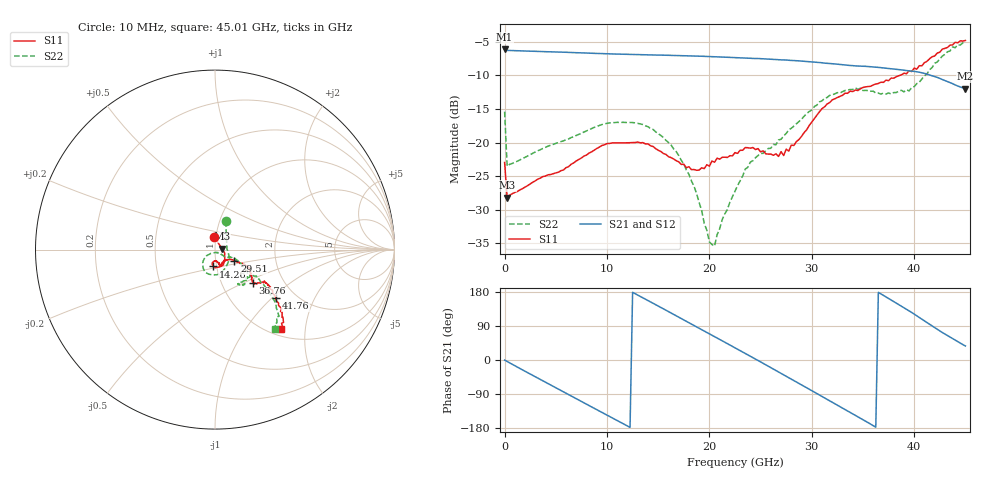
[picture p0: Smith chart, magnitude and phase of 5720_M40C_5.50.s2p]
! Device:  ADRF5720
! Description: 0.5dB LSB GaAs MMIC 6-bit Digital Attenuator
! Frequency:  0.000009 -  40 GHz
! Ports:
!	RF1	= Port 1
!	RF2	= Port 2
! Vdd:  3.3 Volt
! Vss:  -3.3 Volt
! Control:  0/3.3 Volt
! State:  5.50 dB attenuation
! Data:  The device was measured using G-S-G Probes on a matrix board.
!  Data was collected using an calibrated 4 port network analyzer.
!  The reference plane for this measurement is at the launchers.
! Note:  Analog Devices supplies this data as a sample of measured data
!  for this product.  Your particular data for this product may vary.
!  Data was taken at -40 degrees C.
!  Analog Devices reserves the right to change this data at anytime.
# GHZ S DB R 45.0
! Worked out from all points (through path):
!   181 points, 10 MHz to 45.01 GHz, reference 45 ohm
!   highest |S21| = -6.12 dB at 10 MHz (marker M1); lowest = -12.0 dB at 45.01 GHz (marker M2)
!   group delay of S21, straight-line fit = 41.8 ps
!   lowest |S11| = -28.2 dB at 260 MHz (marker M3), VSWR 1.08, Z = 48.6 + j0.56 ohm
!   |S11| at or under -10 dB: start of sweep to 38.61 GHz
!   |S22| runs from -35.4 to -5.1 dB; largest |S21 - S12| = 0.0021
!   S11 on the Smith chart (normalised r, x): 10 MHz: 0.98, +0.14; 14.26 GHz: 0.96, -0.18; 29.51 GHz: 1.23, -0.16; 36.76 GHz: 1.40, -0.57; 41.76 GHz: 1.59, -1.07; 45.01 GHz: 1.11, -1.48
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0.01  -22.97 93.0  -6.12 -0.3  -6.13 -0.3  -15.40 69.3
0.26  -28.19 8.5  -6.28 -4.0  -6.30 -4.0  -23.53 3.5
4.26  -24.80 -19.7  -6.48 -62.5  -6.50 -62.5  -20.53 -32.6
7.76  -22.01 -47.2  -6.66 -113.1  -6.67 -113.1  -18.43 -63.3
11.26  -20.06 -73.9  -6.84 -163.4  -6.86 -163.5  -17.02 -93.3
14.26  -20.48 -95.8  -6.95 153.3  -6.97 153.3  -17.91 -119.3
15.26  -21.32 -99.6  -6.98 138.8  -7.00 138.7  -18.94 -127.5
18.01  -23.60 -94.2  -7.10 98.6  -7.12 98.5  -24.73 -144.2
20.01  -23.52 -80.3  -7.20 69.1  -7.22 69.0  -34.81 -104.8
20.51  -22.93 -78.0  -7.23 61.8  -7.25 61.6  -35.43 -64.5
22.76  -21.61 -75.0  -7.37 28.5  -7.39 28.4  -26.42 -35.3
24.01  -20.84 -69.8  -7.46 9.9  -7.48 9.8  -22.91 -35.9
26.01  -21.72 -58.1  -7.59 -20.0  -7.62 -20.1  -20.86 -27.1
27.26  -21.93 -46.0  -7.70 -38.9  -7.72 -39.0  -19.01 -23.9
29.51  -18.10 -30.1  -7.92 -73.2  -7.95 -73.4  -15.68 -28.0
30.26  -16.45 -27.4  -8.02 -84.8  -8.05 -84.9  -14.64 -31.2
34.01  -12.41 -36.1  -8.55 -142.0  -8.58 -142.1  -12.10 -47.6
36.76  -11.02 -41.7  -8.85 174.5  -8.87 174.3  -12.78 -56.5
37.76  -10.41 -39.5  -9.02 158.4  -9.04 158.2  -12.77 -52.8
39.51  -9.31 -33.3  -9.33 129.8  -9.35 129.6  -12.31 -36.6
41.76  -7.22 -38.5  -10.05 90.0  -10.07 89.8  -8.84 -37.3
45.01  -4.80 -50.6  -11.96 37.0  -11.99 36.8  -5.13 -52.9
